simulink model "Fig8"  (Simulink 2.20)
settings: Solver=ode45  StartTime=0.0  StopTime=15  RelTol=1e-3  AbsTol=1e-6
libraries: simulink x3

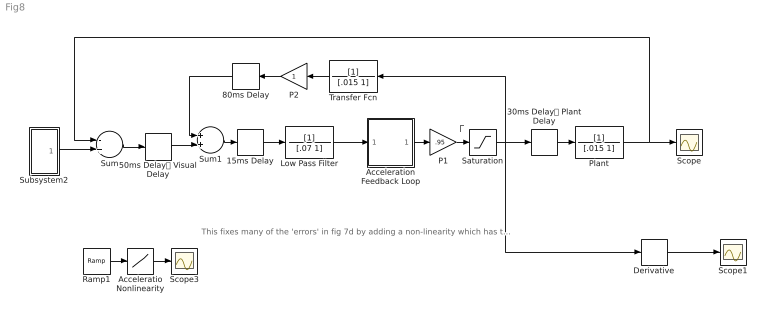
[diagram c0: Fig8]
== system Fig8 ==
  note: 
  note: This fixes many of the 'errors' in fig 7d by adding a non-linearity which has to be either velocity or acceleration. Here an accelleration non-linearity is added (open it up to see it), which reintroduces oscillations and produces a non-linear dependence of initial pursuit velocity on initial silp velocity.
  15ms Delay : TransportDelay  DelayTime=.015  InitialInput=0  BufferSize=1024
  30ms Delay Plant Delay : TransportDelay  DelayTime=.030  InitialInput=0  BufferSize=1024
  50ms Delay Visual Delay : TransportDelay  DelayTime=.050  InitialInput=0  BufferSize=1024
  80ms Delay : TransportDelay  Orientation=left  DelayTime=.08  InitialInput=0  BufferSize=1024
  Acceleratio Nonlinearity : Lookup  InputValues=[-100:100]  OutputValues=[-40+(-100:-5)*5 (-4:-1)*15 (0:4)*15 40+(5:100)*5]
  Acceleration Feedback Loop : Subsystem
  Derivative : Derivative
  Low Pass Filter : TransferFcn  Numerator=[1]  Denominator=[.07 1]
  P1 : Gain  Gain=.95
  P2 : Gain  Orientation=left  Gain=1
  Plant : TransferFcn  Numerator=[1]  Denominator=[.015 1]
  Ramp1 : simulink/Sources/Ramp  slope=1  start=0  X0=-100
  Saturation : Saturate  UpperLimit=90  LowerLimit=-90
  Scope : Scope
  Scope1 : Scope
  Scope3 : Scope
  Subsystem2 : Subsystem
  Sum : Sum  Inputs=-+
  Sum1 : Sum  Inputs=++
  Transfer Fcn : TransferFcn  Orientation=left  Numerator=[1]  Denominator=[.015 1]
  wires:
  Plant/1 -> Scope/1, Sum/1
  15ms Delay/1 -> Low Pass Filter/1
  Sum/1 -> 50ms Delay Visual Delay/1
  50ms Delay Visual Delay/1 -> Sum1/2
  30ms Delay Plant Delay/1 -> Plant/1
  Derivative/1 -> Scope1/1
  80ms Delay/1 -> Sum1/1
  Transfer Fcn/1 -> P2/1
  P2/1 -> 80ms Delay/1
  Sum1/1 -> 15ms Delay/1
  Ramp1/1 -> Acceleratio Nonlinearity/1
  Acceleratio Nonlinearity/1 -> Scope3/1
  Low Pass Filter/1 -> Acceleration Feedback Loop/1(In1)
  Acceleration Feedback Loop/1(Out1) -> P1/1
  P1/1 -> Saturation/1
  Saturation/1 -> 30ms Delay Plant Delay/1, Transfer Fcn/1, Derivative/1
  Subsystem2/1(Out1) -> Sum/2

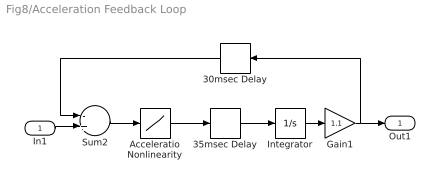
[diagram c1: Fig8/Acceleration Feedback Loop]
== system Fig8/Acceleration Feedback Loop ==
  In1 : Inport  Port=1  PortWidth=-1  SampleTime=-1
  30msec Delay : TransportDelay  Orientation=left  DelayTime=.030  InitialInput=0  BufferSize=1024
  35msec Delay : TransportDelay  DelayTime=.035  InitialInput=0  BufferSize=1024
  Acceleratio Nonlinearity : Lookup  InputValues=[-100:100]  OutputValues=[-40+(-100:-5)*5 (-4:-1)*15 (0:4)*15 40+(5:100)*5]
  Gain1 : Gain  Gain=1.1
  Integrator : Integrator  ExternalReset=none  InitialConditionSource=internal  InitialCondition=0  LimitOutput=off  UpperSaturationLimit=inf  LowerSaturationLimit=-inf  ShowSaturationPort=off  ShowStatePort=off  AbsoluteTolerance=auto
  Sum2 : Sum  Inputs=-+
  Out1 : Outport  Port=1  InitialOutput=0
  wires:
  Integrator/1 -> Gain1/1
  35msec Delay/1 -> Integrator/1
  Gain1/1 -> 30msec Delay/1, Out1/1
  In1/1 -> Sum2/2
  Sum2/1 -> Acceleratio Nonlinearity/1
  Acceleratio Nonlinearity/1 -> 35msec Delay/1
  30msec Delay/1 -> Sum2/1

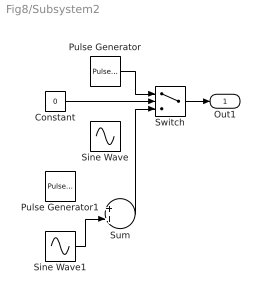
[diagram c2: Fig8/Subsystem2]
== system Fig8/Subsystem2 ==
  Constant : Constant  Value=0
  Pulse Generator : simulink/Sources/Pulse Generator  period=100  duty=50  amplitude=20  start=0
  Pulse Generator1 : simulink/Sources/Pulse Generator  period=100  duty=50  amplitude=20  start=0
  Sine Wave : Sin  Amplitude=10  Frequency=10*pi*2  Phase=0  SampleTime=0
  Sine Wave1 : Sin  Amplitude=8  Frequency=6*pi*2  Phase=0  SampleTime=0
  Sum : Sum  Inputs=++
  Switch : Switch  Threshold=1
  Out1 : Outport  Port=1  InitialOutput=0
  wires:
  Pulse Generator/1 -> Switch/1
  Constant/1 -> Switch/2
  Switch/1 -> Out1/1
  Sine Wave1/1 -> Sum/2
  Sum/1 -> Switch/3
